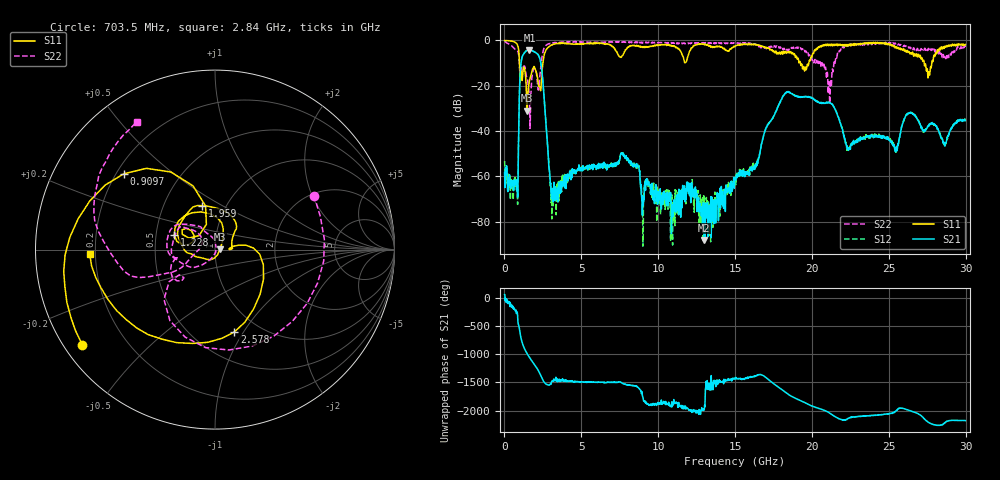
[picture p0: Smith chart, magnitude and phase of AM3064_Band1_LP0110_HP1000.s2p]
# Hz S DB R 50.0
!freq dBS11 angS11 dBS21 angS21 dBS12 angS12 dBS22 angS22
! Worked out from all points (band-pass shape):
!   1600 points, 10 MHz to 29.98 GHz, reference 50 ohm
!   highest |S21| = -4.21 dB at 1.622 GHz (marker M1); lowest = -88.1 dB at 13 GHz (marker M2)
!   |S21| within 3 dB of the highest: 1.156 GHz to 2.255 GHz (1.099 GHz wide, 64.4 % of centre)
!   lowest |S11| = -31.0 dB at 1.453 GHz (marker M3), VSWR 1.06, Z = 52.9 + j0.173 ohm
!   |S11| at or under -10 dB: 973.9 MHz to 2.503 GHz (1.529 GHz wide, 88 % of centre); 19.25 GHz to 19.79 GHz (544.2 MHz wide, 2.79 % of centre); 27.3 GHz to 27.8 GHz (495.8 MHz wide, 1.8 % of centre)
!   |S22| runs from -38.8 to -0.4 dB; largest |S21 - S12| = 0.0073
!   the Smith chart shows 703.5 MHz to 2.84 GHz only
!   S11 on the Smith chart (normalised r, x): 703.5 MHz: 0.05, -0.32; 909.7 MHz: 0.23, +0.34; 1.228 GHz: 0.62, +0.11; 1.959 GHz: 0.77, +0.41; 2.578 GHz: 0.77, -0.91; 2.84 GHz: 0.18, -0.02
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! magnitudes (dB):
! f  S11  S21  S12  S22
! 10 MHz  0.0  -58.3  -53.2  -0.4
! 703.5 MHz  -0.8  -63.6  -60.6  -4.0
! 909.7 MHz  -3.6  -46.8  -47.3  -5.8
! 1.228 GHz  -12.4  -6.2  -6.1  -11.7
! 1.453 GHz  -31.0  -4.4  -4.4  -16.4
! 1.622 GHz  -18.0  -4.2  -4.2  -26.2
! 1.959 GHz  -11.9  -5.1  -5.1  -12.4
! 2.578 GHz  -6.5  -25.1  -25.2  -3.2
! 2.84 GHz  -3.1  -49.8  -50.1  -1.6
! 3.215 GHz  -1.6  -62.5  -66.8  -1.0
! 5.015 GHz  -1.4  -57.0  -56.4  -0.6
! 7.714 GHz  -6.4  -50.8  -49.2  -0.8
! 10 GHz  -2.0  -71.5  -70.1  -1.0
! 13 GHz  -1.9  -88.1  -71.0  -1.2
! 15 GHz  -2.5  -60.5  -60.9  -1.3
! 18.25 GHz  -5.0  -23.3  -23.4  -4.4
! 19.99 GHz  -7.3  -25.4  -25.4  -8.2
! 21.15 GHz  -1.7  -27.5  -27.6  -27.8
! 22.35 GHz  -1.8  -47.6  -48.4  -2.2
! 25 GHz  -1.5  -43.8  -43.6  -1.3
! 27.56 GHz  -16.4  -37.8  -37.7  -3.7
! 29.98 GHz  -1.8  -35.3  -35.2  -2.9
